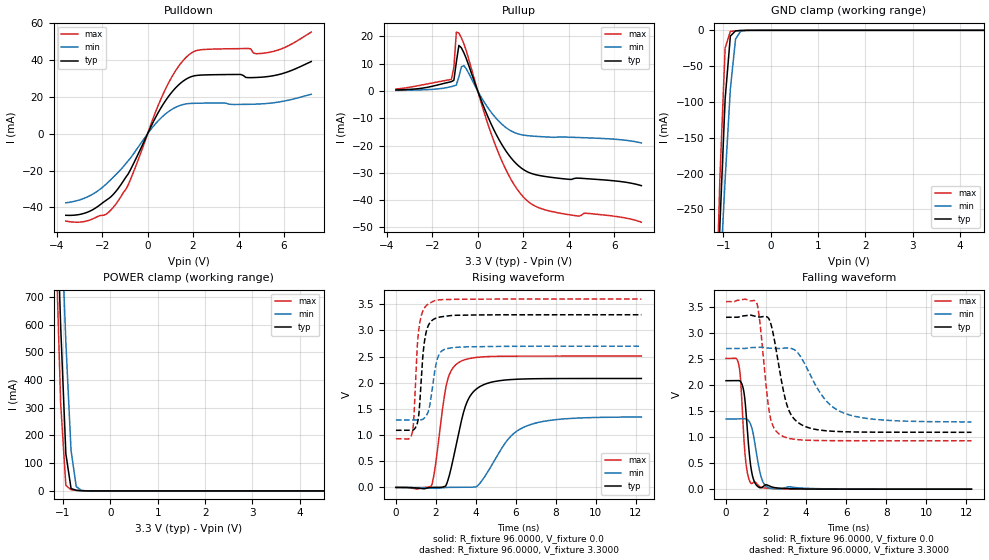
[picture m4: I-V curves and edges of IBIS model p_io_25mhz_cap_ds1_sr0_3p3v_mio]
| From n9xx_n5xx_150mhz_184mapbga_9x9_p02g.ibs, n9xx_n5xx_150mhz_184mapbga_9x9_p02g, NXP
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[Model] p_io_25mhz_cap_ds1_sr0_3p3v_mio
|   Model p_io_25mhz_cap_ds1_sr0_3p3v_mio
| This model was characterised for following simulation conditions:
| External (pad) voltage:
|   - Typ: 3.3V,   - Min: 2.7V,   - Max: 3.6V
| Library cells for typ/min/max conditions are connected as defined below:
|  pad - External Pad
|  ipp_do_lv - Core Input
|  ipp_obe_lv - Output Buffer Enable
|  IOGC - NC
|  REFH3V3 - REFH3V3
|  REFL3V3 - REFL3V3
|  ZI - NC
|  abut_ncal_vddio[1] - vddio
|  abut_ncal_vddio[2] - vddio
|  abut_ncal_vddio[3] - vssio
|  abut_ncal_vddio[4] - vddio
|  abut_ncal_vddio[5] - vddio
|  abut_ncal_vddio[6] - vssio
|  abut_pcal_vddio[1] - vssio
|  abut_pcal_vddio[2] - vssio
|  abut_pcal_vddio[3] - vddio
|  abut_pcal_vddio[4] - vssio
|  abut_pcal_vddio[5] - vssio
|  abut_pcal_vddio[6] - vddio
|  ipp_do_1p8v - ipp_do_1p8v
|  ipp_dse_lv - vdd_lv
|  ipp_eftd_lv - NC
|  ipp_ina_mux_vddio - NC
|  ipp_ina_mux_vddio[0] - NC
|  ipp_ina_mux_vddio[1] - NC
|  ipp_ina_r0_vddio - NC
|  ipp_ina_r0a_vddio - NC
|  ipp_ina_r0b_vddio - NC
|  ipp_ina_r0c_vddio - NC
|  ipp_ina_r0d_vddio - NC
|  ipp_ina_r0e_vddio - NC
|  ipp_ina_r0f_vddio - NC
|  ipp_ina_r300_vddio - NC
|  ipp_ina_r300a_vddio - NC
|  ipp_ina_r300b_vddio - NC
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Model_type I/O
Polarity   Non-Inverting
Enable   Active-High
Vinl =   0.9900V
Vinh =   2.3100V
Vmeas =  1.6500V
Cref =   30.0000pF
Rref =   1.0000M
Vref =   3.3000V
C_comp   1.2811pF   1.2304pF   1.3502pF
|C_comp_pullup   0.5376pF   0.5687pF   0.5163pF
|C_comp_pulldown   0.6574pF   0.6940pF   0.6283pF
[Model Spec]
| variable   typ   min   max
Vinh   2.3100V   1.8900V   2.5200V
Vinl   0.9900V   0.8100V   1.0800V
[Temperature Range]   25.0000   0.1250k   -40.0000
[Voltage Range]   3.3000V   2.7000V   3.6000V
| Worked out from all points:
|   slope of the pulldown table from 0 to 0.495 V, typ, clamps not added: 40.8 ohm
|   slope of the pullup table from 0 to 0.495 V, typ, clamps not added: 47.8 ohm
|   GND clamp passes 1 mA (typ) near -0.74 V on its own axis
|   POWER clamp passes 1 mA (typ) near -0.62 V on its own axis
|   rising waveform, R_fixture 96.0000, V_fixture 0.0: 20-80 % time 805ps typ, 1.51ns min, 547ps max; typ from 0 V to 2.08 V
|   rising waveform, R_fixture 96.0000, V_fixture 3.3000: 20-80 % time 277ps typ, 351ps min, 246ps max; typ from 1.09 V to 3.3 V
|   falling waveform, R_fixture 96.0000, V_fixture 0.0: 20-80 % time 287ps typ, 380ps min, 249ps max; typ from 2.08 V to 0 V
|   falling waveform, R_fixture 96.0000, V_fixture 3.3000: 20-80 % time 699ps typ, 1.44ns min, 438ps max; typ from 3.3 V to 1.09 V
[Pulldown]
|Voltage   I(typ)   I(min)   I(max)
-3.6V     -44.37mA   -37.58mA   -47.51mA
-2.5V     -41.88mA   -33.45mA   -46.76mA
-1.84V    -36.35mA   -27.58mA   -43.93mA
-1.4V     -31.44mA   -22.29mA   -38.35mA
-850mV    -21.79mA   -14.63mA   -27.74mA
800mV     18.21mA    10.89mA    24.66mA
1.35V     26.41mA    15.03mA    36.45mA
1.9V      30.96mA    16.49mA    43.73mA
4.43V     30.52mA    16mA       46.39mA
4.76V     30.6mA     16.11mA    43.53mA
5.31V     31.15mA    16.53mA    44.19mA
7.2V      39.28mA    21.46mA    55.3mA
[Pullup]
|Voltage   I(typ)   I(min)   I(max)
-3.6V     375uA      207.1uA    721uA
-1.16V    3.419mA    1.608mA    4.218mA
-1.05V    3.929mA    1.825mA    8.684mA
-940mV    10.66mA    2.209mA    21.58mA
-830mV    16.7mA     5.227mA    21.23mA
-720mV    15.82mA    8.86mA     19.48mA
-610mV    14mA       9.299mA    17.3mA
820mV     -16.02mA   -10.13mA   -20.76mA
1.48V     -24.66mA   -14.68mA   -32.62mA
2.03V     -28.88mA   -16.19mA   -39.03mA
3.35V     -31.76mA   -16.97mA   -44.31mA
7.2V      -34.67mA   -19.04mA   -48.06mA
[GND_clamp]
|Voltage   I(typ)   I(min)   I(max)
-3.6V     -5.309A    -4.128A    -6.876A
-1.18V    -466mA     -495.4mA   -458.9mA
-1.07V    -271.1mA   -348.5mA   -204.6mA
-960mV    -95.65mA   -207.9mA   -24.72mA
-850mV    -8.088mA   -81.85mA   -1.461mA
-740mV    -716.3uA   -12.13mA   -715.9uA
-630mV    -272.3uA   -921.7uA   -303uA
-300mV    -444.9nA   -2.656uA   -94.82nA
7.2V      0A         0A         0A
[POWER_clamp]
|Voltage   I(typ)   I(min)   I(max)
-3.6V     14.48A     12.95A     16.35A
-1.16V    1.177A     1.535A     951.2mA
-1.05V    598.4mA    1.032A     318mA
-940mV    134.2mA    537.3mA    20.05mA
-830mV    8.719mA    145.4mA    4.267mA
-720mV    2.135mA    15.38mA    2.236mA
-610mV    852.8uA    1.854mA    844.7uA
7.2V      0A         0A         0A
[Ramp]
| variable   typ   min   max
dV/dt_r  1.2493/0.8047n   0.8077/1.5069n   1.5061/0.5473n
dV/dt_f  1.3249/0.6986n   0.8456/1.4368n   1.6024/0.4383n
R_load = 96.0000
[Rising Waveform]
R_fixture= 96.0000
V_fixture= 0.0
V_fixture_min= 0.0
V_fixture_max= 0.0
|time   V(typ)   V(min)   V(max)
0s        3.103nV    104.7nV    10.53nV
1.774ns   241.8uV    -13.69mV   32.51mV
1.946ns   1.944mV    -17.02mV   346.1mV
2.55ns    81.48mV    155.7uV    2.006V
3.243ns   1.224V     1.206mV    2.41V
3.585ns   1.659V     924.1uV    2.456V
4.125ns   1.91V      46.67mV    2.489V
5.554ns   2.056V     895.1mV    2.508V
6.502ns   2.074V     1.17V      2.51V
12.27ns   2.082V     1.346V     2.51V
[Rising Waveform]
R_fixture= 96.0000
V_fixture= 3.3000
V_fixture_min= 2.7000
V_fixture_max= 3.6000
|time   V(typ)   V(min)   V(max)
0s        1.092V     1.289V     929.3mV
814.5ps   1.091V     1.289V     1.041V
895ps     1.105V     1.289V     1.326V
1.065ns   1.221V     1.289V     2.691V
1.166ns   1.484V     1.288V     3.08V
1.397ns   2.701V     1.317V     3.412V
1.67ns    3.131V     1.529V     3.518V
2.066ns   3.244V     2.449V     3.581V
2.492ns   3.273V     2.646V     3.591V
12.27ns   3.3V       2.7V       3.6V
[Falling Waveform]
R_fixture= 96.0000
V_fixture= 0.0
V_fixture_min= 0.0
V_fixture_max= 0.0
|time   V(typ)   V(min)   V(max)
0s        2.082V     1.348V     2.51V
501.4ps   2.082V     1.348V     2.511V
652.9ps   2.084V     1.348V     2.358V
736.3ps   2.061V     1.348V     2.054V
970ps     1.609V     1.35V      584.2mV
1.256ns   384.4mV    1.216V     110.7mV
1.45ns    116mV      861.1mV    136.9mV
1.76ns    27.96mV    227.7mV    35.18mV
2.166ns   60.69mV    21.9mV     15.26mV
12.27ns   223.4nV    15.76uV    31.21nV
[Falling Waveform]
R_fixture= 96.0000
V_fixture= 3.3000
V_fixture_min= 2.7000
V_fixture_max= 3.6000
|time   V(typ)   V(min)   V(max)
0s        3.3V       2.7V       3.6V
1.528ns   3.312V     2.723V     3.58V
1.675ns   3.304V     2.727V     3.26V
2.172ns   3.248V     2.707V     1.458V
2.772ns   2.075V     2.703V     1.028V
3.104ns   1.547V     2.709V     979.3mV
3.588ns   1.283V     2.618V     950.3mV
4.875ns   1.126V     1.758V     932.5mV
5.883ns   1.103V     1.462V     930.2mV
12.27ns   1.092V     1.291V     929.3mV
